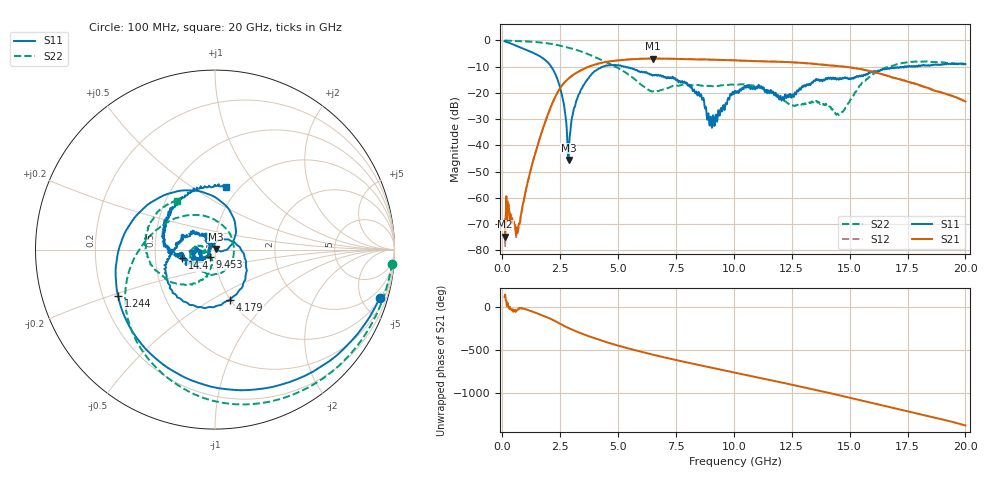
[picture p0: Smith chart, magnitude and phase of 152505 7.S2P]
!  2-Port S-parameters saved by WinCal
! VAR MeasName=S-Parameters (CALIBRATED_DATA) read from VNA (N5230C)
! VAR MeasDate=4/10/2015 9:29:04 AM
! VAR NAME=152505 7
! VAR FILENAME=152505 7.S2P
! VAR DATE=4/10/2015 9:29:04 AM
! VAR PHYS_PORTS=1,2
# Hz S DB R 50
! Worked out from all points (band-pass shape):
!   801 points, 100 MHz to 20 GHz, reference 50 ohm
!   highest |S21| = -6.96 dB at 6.493 GHz (marker M1); lowest = -74.8 dB at 124.9 MHz (marker M2)
!   |S21| within 3 dB of the highest: 3.767 GHz to 14.65 GHz (10.88 GHz wide, 118 % of centre)
!   lowest |S11| = -45.6 dB at 2.861 GHz (marker M3), VSWR 1.01, Z = 50.3 + j0.394 ohm
!   |S11| at or under -10 dB: 2.109 GHz to 4.358 GHz (2.249 GHz wide, 69.5 % of centre); 5.234 GHz to 17.37 GHz (12.14 GHz wide, 107 % of centre); 17.40068 GHz to 17.46145 GHz (60.78 MHz wide, 0.349 % of centre)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
!   |S22| runs from -28.5 to -0.1 dB; largest |S21 - S12| = 0.0065
!   S11 on the Smith chart (normalised r, x): 100 MHz: 1.06, -6.80; 1.244 GHz: 0.26, -0.21; 4.179 GHz: 1.00, -0.61; 9.453 GHz: 0.94, -0.08; 14.4 GHz: 0.69, -0.07; 20 GHz: 0.87, +0.69
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1e8  -0.38 -16.3  -68.76 112.0  -67.83 133.4  -0.08 -4.5
1.24875e8  -0.47 -20.0  -74.77 140.4  -78.38 88.2  -0.10 -5.5
2.74125e8  -0.92 -41.0  -62.73 -10.3  -62.94 -8.2  -0.17 -11.5
6.72125e8  -2.33 -91.3  -72.92 -33.6  -72.08 -31.8  -0.32 -27.3
1.24425e9  -4.45 -154.4  -48.72 -52.7  -48.67 -52.3  -0.57 -50.4
1.866125e9  -7.62 133.4  -30.75 -115.9  -30.76 -115.9  -1.06 -76.5
2.313875e9  -13.34 64.0  -21.09 -173.4  -21.11 -173.2  -1.71 -96.2
2.861125e9  -45.62 48.3  -14.58 110.5  -14.56 110.8  -2.84 -119.7
3.43325e9  -18.39 15.7  -11.30 45.5  -11.28 45.8  -4.36 -144.6
4.1795e9  -10.69 -73.1  -8.82 -26.0  -8.80 -25.8  -7.12 -176.1
5.1745e9  -9.87 -144.0  -7.53 -107.1  -7.50 -107.2  -11.47 137.0
6.492875e9  -13.48 174.7  -6.96 161.1  -6.97 161.1  -19.49 13.7
6.741625e9  -13.15 170.7  -6.99 145.2  -6.96 144.8  -19.30 -18.1
7.935625e9  -16.42 138.7  -7.21 72.3  -7.17 72.5  -16.86 -104.6
8.9555e9  -32.46 112.5  -7.39 12.8  -7.40 13.0  -17.40 -133.2
9.453e9  -25.79 -126.4  -7.49 -15.6  -7.51 -15.6  -17.21 -139.5
1.005e10  -19.24 -142.4  -7.65 -49.6  -7.65 -49.7  -16.87 -151.7
1.196538e10  -22.54 -175.4  -8.19 -157.9  -8.19 -157.7  -22.06 166.2
1.338325e10  -16.14 -151.3  -8.96 118.5  -8.90 118.6  -23.35 -164.3
1.440312e10  -14.47 -165.5  -9.76 57.5  -9.80 56.7  -28.15 -157.1
1.669162e10  -10.85 171.0  -13.68 -88.8  -13.76 -89.9  -10.03 -147.1
2e10  -9.07 80.2  -23.34 56.4  -23.35 56.9  -9.22 128.1
